PROGRAM MAIN
VAR
	p07_ST_motor_0: p07_ST_motor;
	buttonLeft: BOOL;
	buttonRight: BOOL;
	motorMovement: BOOL;
	motorDirection: BOOL;
	FB_materialTracking: p08_ST_materialTracking;
END_VAR

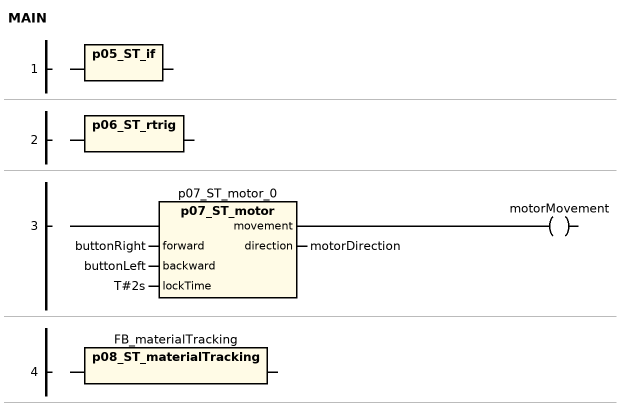
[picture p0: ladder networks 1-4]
// NETWORK 1
p05_ST_if();

// NETWORK 2
p06_ST_rtrig();

// NETWORK 3
p07_ST_motor_0(forward := buttonRight, backward := buttonLeft, lockTime := T#2s, direction => motorDirection); // p07_ST_motor
motorMovement := p07_ST_motor_0.movement;

// NETWORK 4
FB_materialTracking(); // p08_ST_materialTracking

END_PROGRAM
